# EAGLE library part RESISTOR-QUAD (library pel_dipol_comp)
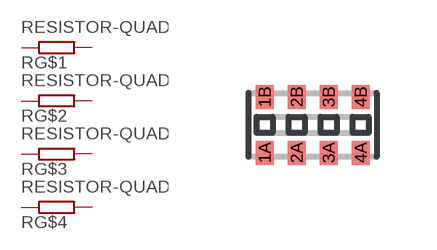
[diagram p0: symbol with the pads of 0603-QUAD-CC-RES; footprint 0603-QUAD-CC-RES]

Designator prefix R; gates G$1=RESISTOR G$2=RESISTOR G$3=RESISTOR G$4=RESISTOR

## RESISTOR-QUAD-0603  [0603-QUAD-CC-RES]
1A  G$1:1  pas
1B  G$1:2  pas
2A  G$2:1  pas
2B  G$2:2  pas
3A  G$3:1  pas
3B  G$3:2  pas
4A  G$4:1  pas
4B  G$4:2  pas

## Footprint 0603-QUAD-CC-RES (pad centres in mm)
Concave 4 resistor array
smd 0.45 x 0.6: 1A -1.2,-0.7; 1B -1.2,0.7; 2A -0.4,-0.7; 2B -0.4,0.7; 3A 0.4,-0.7; 3B 0.4,0.7; 4A 1.2,-0.7; 4B 1.2,0.7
